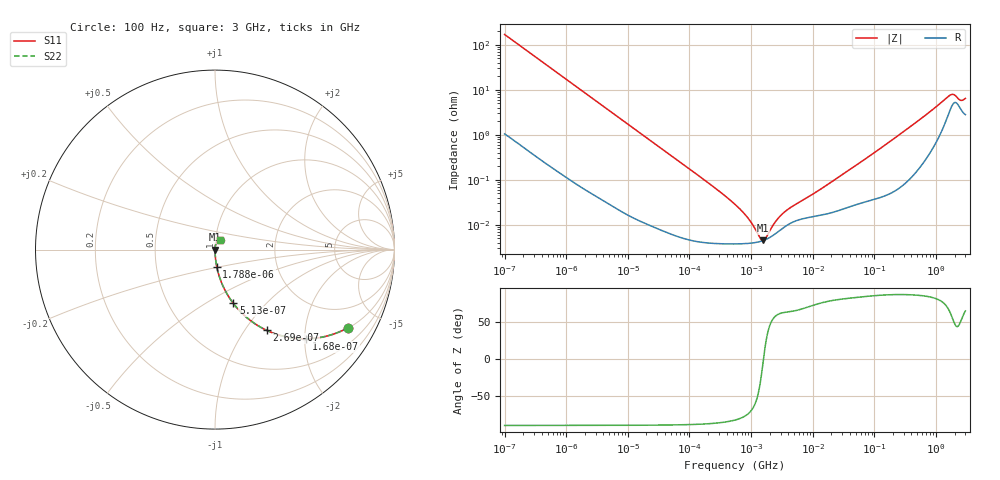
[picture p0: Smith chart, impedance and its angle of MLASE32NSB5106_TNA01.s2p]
! MLASE32NSB5106_TNA01  S-PARAMETER MODEL  ( Standard Model )
! Model Generated by TAIYO YUDEN Corporation (http://www.ty-top.com)
! Version 1.0
! TAIYO YUDEN Control No. 220601
! Copyright(c) 2009 TAIYO YUDEN CO.,LTD. All Rights Reserved.
! Product Description (link to TY-COMPAS)
! https://ds.yuden.co.jp/TYCOMPAS/or/detail?pn=MLASE32NSB5106KTNA01&u=M
! Products Name : Multilayer Ceramic Capacitors
! Characteristics :
!  Capacitance : 10 [uF] , Rated Voltage : 16 [V] , TCC : X5R
!  Case Size : 3.2 x 2.5 / 0.126 x 0.098 [mm/inch] , Thickness : 1.9 / 0.075 [mm/inch]
!  (Conditions: Temperature = 25 [degC] , DC Bias Voltage = 0 [V])
! External Node Assignments :
!  1  o---| |---o  2
! GND o---------o GND
! Frequency Range : 100Hz  -  3GHz  [ 401 STEP ]
# MHZ S RI R 50
! Freq[MHz].  S11 Real  S11 Imag  S21 Real  S21 Imag  S12 Real  S12 Imag  S22 Real  S22 Imag
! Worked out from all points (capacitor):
!   401 points, 100 Hz to 3 GHz, reference 50 ohm
!   read as one part in series: C = 9.34 uF near 109 Hz
!   lowest |Z| = 4.51 mohm at 1.539 MHz (marker M1)
!   series resonance near 1.59 MHz, so ESL is about 1.1 nH
!   S11 on the Smith chart (normalised r, x): 100 Hz: 1.02, -3.41; 168 Hz: 1.01, -2.04; 269 Hz: 1.01, -1.27; 513 Hz: 1.00, -0.67; 1.788 kHz: 1.00, -0.19; 3 GHz: 1.06, +0.12
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0.0001  0.7422 -0.4343  0.2578 0.4343  0.2578 0.4343  0.7422 -0.4343
0.000168  0.5089 -0.4968  0.4911 0.4968  0.4911 0.4968  0.5089 -0.4968
0.000269  0.2888 -0.4501  0.7112 0.4501  0.7112 0.4501  0.2888 -0.4501
0.000513  0.1019 -0.2993  0.8981 0.2993  0.8981 0.2993  0.1019 -0.2993
0.00086  0.0395 -0.1915  0.9605 0.1915  0.9605 0.1915  0.0395 -0.1915
0.001788  0.00985 -0.0953  0.9902 0.0953  0.9902 0.0953  0.00985 -0.0953
0.005476  0.00126 -0.0316  0.9987 0.0316  0.9987 0.0316  0.00126 -0.0316
0.031977  0.00011 -0.00546  0.9999 0.00546  0.9999 0.00546  0.00011 -0.00546
0.231582  3.96e-05 -0.000745  1 0.000745  1 0.000745  3.96e-05 -0.000745
0.547723  3.8e-05 -0.000284  1 0.000284  1 0.000284  3.8e-05 -0.000284
0.740304  3.83e-05 -0.000187  1 0.000187  1 0.000187  3.83e-05 -0.000187
1.044606  3.97e-05 -9.66e-05  1 9.66e-05  1 9.66e-05  3.97e-05 -9.66e-05
1.138514  4.03e-05 -7.6e-05  1 7.6e-05  1 7.6e-05  4.03e-05 -7.6e-05
1.53882  4.45e-05 -7.27e-06  1 7.27e-06  1 7.27e-06  4.45e-05 -7.27e-06
2.266852  5.84e-05 7.9e-05  0.9999 -7.9e-05  0.9999 -7.9e-05  5.84e-05 7.9e-05
3.79959  9.78e-05 0.00019  0.9999 -0.00019  0.9999 -0.00019  9.78e-05 0.00019
9.794414  0.000151 0.000449  0.9998 -0.000449  0.9998 -0.000449  0.000151 0.000449
175.1444  0.000536 0.00696  0.9995 -0.00696  0.9995 -0.00696  0.000536 0.00696
1642.185  0.0351 0.0628  0.9649 -0.0628  0.9649 -0.0628  0.0351 0.0628
1950.712  0.0517 0.0539  0.9483 -0.0539  0.9483 -0.0539  0.0517 0.0539
2525.516  0.0376 0.0419  0.9624 -0.0419  0.9624 -0.0419  0.0376 0.0419
3000  0.0306 0.055  0.9694 -0.055  0.9694 -0.055  0.0306 0.055
